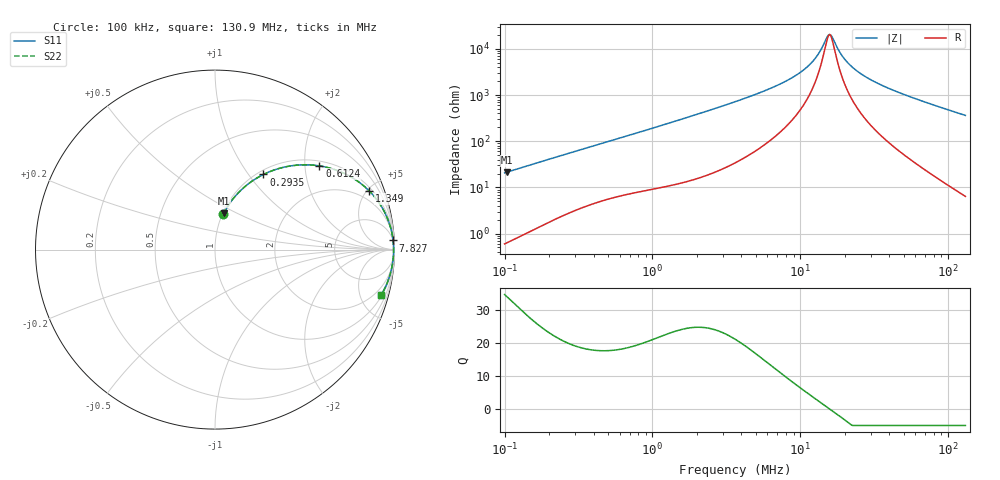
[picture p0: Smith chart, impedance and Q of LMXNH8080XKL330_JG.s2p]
! LMXNH8080XKL330_JG  S-PARAMETER MODEL  ( General Type )
! Model Generated by TAIYO YUDEN Corporation (http://www.ty-top.com)
! Version 1.0
! TAIYO YUDEN Control No. 191025NI43SB-FBB
! Copyright(c) 2019 TAIYO YUDEN CO.,LTD. All Rights Reserved.
! Product Description (link to TY-COMPAS)
! https://ds.yuden.co.jp/TYCOMPAS/or/detail?pn=LMXNH8080XKL330MJG&u=M
! Products Name : Inductors
! Characteristics :
!  Inductance : 33 uH , SRF(min) : 13 MHz , DC Resistance(max) : 0.156 Ohm
!  Rated Current : Saturation :1300 mA , Temp Rise : 1500 mA
!  Case Size : 8.0 x 8.0 / 0.315 x 0.315 [mm/inch] , Thickness : 3 / 0.118 [mm/inch]
!  (Conditions: Temperature = 25 degC , DC Bias Current/Voltage = 0A / 0V)
! External Node Assignments :
!  1  o---GGG---o  2
! GND o---------o GND
! Frequency Range : 0.1MHz  -  130.914307MHz  [ 402 STEP ]
# MHz S RI R 50
! Freq[MHz].  S11 Real  S11 Imag  S21 Real  S21 Imag  S12 Real  S12 Imag  S22 Real  S22 Imag
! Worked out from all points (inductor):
!   401 points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, 100 kHz to 130.9 MHz, reference 50 ohm
!   read as one part in series: L = 32.8 uH near 103.7 kHz
!   highest Q = 34 at 103.7 kHz (marker M1), where L = 32.9 uH
!   self-resonance near 15.76 MHz
!   S11 on the Smith chart (normalised r, x): 100 kHz: 1.01, +0.41; 293.5 kHz: 1.06, +1.18; 612.4 kHz: 1.13, +2.38; 1.349 MHz: 1.22, +5.14; 7.827 MHz: 5, +39; 130.9 MHz: 1.13, -7.25
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0.1  0.0462 0.196  0.9538 -0.196  0.9538 -0.196  0.0462 0.196
0.103654  0.0493 0.2023  0.9507 -0.2023  0.9507 -0.2023  0.0493 0.2023
0.177566  0.1266 0.3129  0.8734 -0.3129  0.8734 -0.3129  0.1266 0.3129
0.293459  0.2694 0.4184  0.7306 -0.4184  0.7306 -0.4184  0.2694 0.4184
0.332733  0.3167 0.4389  0.6833 -0.4389  0.6833 -0.4389  0.3167 0.4389
0.612406  0.5821 0.4664  0.4179 -0.4664  0.4179 -0.4664  0.5821 0.4664
1.10711  0.8065 0.3727  0.1935 -0.3727  0.1935 -0.3727  0.8065 0.3727
1.348677  0.8583 0.3278  0.1417 -0.3278  0.1417 -0.3278  0.8583 0.3278
2.112125  0.9344 0.2283  0.0656 -0.2283  0.0656 -0.2283  0.9344 0.2283
3.683715  0.9755 0.1324  0.0245 -0.1324  0.0245 -0.1324  0.9755 0.1324
7.826537  0.9923 0.0507  0.00772 -0.0507  0.00772 -0.0507  0.9923 0.0507
10.06153  0.994 0.0311  0.00595 -0.0311  0.00595 -0.0311  0.994 0.0311
12.03896  0.9948 0.0184  0.00524 -0.0184  0.00524 -0.0184  0.9948 0.0184
13.40737  0.995 0.011  0.00499 -0.011  0.00499 -0.011  0.995 0.011
15.20166  0.9952 0.00256  0.00485 -0.00256  0.00485 -0.00256  0.9952 0.00256
16.04237  0.9952 -0.00103  0.00483 0.00103  0.00483 0.00103  0.9952 -0.00103
19.19522  0.995 -0.0131  0.00498 0.0131  0.00498 0.0131  0.995 -0.0131
22.55928  0.9946 -0.0243  0.00538 0.0243  0.00538 0.0243  0.9946 -0.0243
28.48573  0.9935 -0.0417  0.00652 0.0417  0.00652 0.0417  0.9935 -0.0417
40.05754  0.9901 -0.0712  0.00988 0.0712  0.00988 0.0712  0.9901 -0.0712
68.62119  0.9766 -0.1349  0.0234 0.1349  0.0234 0.1349  0.9766 -0.1349
130.9143  0.9255 -0.2538  0.0745 0.2538  0.0745 0.2538  0.9255 -0.2538
